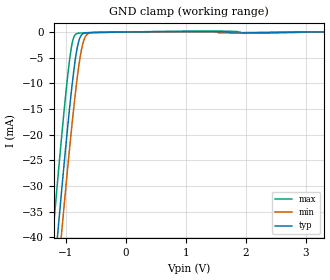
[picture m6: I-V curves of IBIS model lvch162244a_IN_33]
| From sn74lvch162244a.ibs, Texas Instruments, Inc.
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[Model]   lvch162244a_IN_33
Model_type  Input
Vinl=0.8
Vinh=2.0
| variable   typ   min   max
C_comp   3.34pF   2.56pF   4.57pF
[Temperature Range]   40   100   -40
| Ambient temperature   25   85   -40
[Voltage range]   3.3   3   3.6
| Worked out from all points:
|   GND clamp passes 1 mA (typ) near -0.76 V on its own axis
[GND Clamp]
| lvch162244a_IN_33
|   Voltage   I(typ)   I(min)   I(max)
-5.5V     -656.9mA   -663.6mA   -648.6mA
-1.225V   -51.21mA   -59.43mA   -40.69mA
-1.195V   -47.22mA   -55.45mA   -36.68mA
-1.145V   -40.63mA   -48.86mA   -30.08mA
-1.08V    -32.22mA   -40.43mA   -21.71mA
-1.06V    -29.67mA   -37.87mA   -19.2mA
-965mV    -18.04mA   -26.02mA   -8.161mA
-885mV    -9.27mA    -16.68mA   -1.724mA
-775mV    -1.431mA   -5.931mA   -215.8uA
-715mV    -331.4uA   -2.217mA   -184.8uA
-640mV    -125.1uA   -413.3uA   -161.8uA
3.3V      9.604pA    40.59nA    -142.9nA
